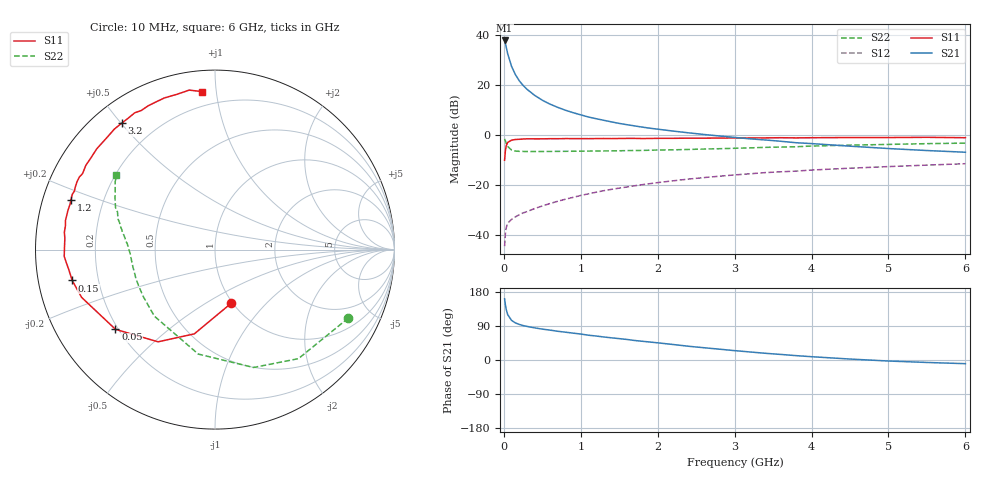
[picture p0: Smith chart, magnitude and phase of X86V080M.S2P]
! SIEMENS Small Signal Semiconductors
! BFP136W
! Si NPN RF Bipolar Junction Transistor in SOT343
! VCE = 6 V  IC = 80 mA
! Common Emitter S-Parameters:  September  1994
# GHz  S  MA  R  50
!  f  S11  S21  S12  S22
! GHz  MAG  ANG  MAG  ANG  MAG  ANG  MAG  ANG
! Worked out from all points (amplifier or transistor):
!   40 points, 10 MHz to 6 GHz, reference 50 ohm
!   highest |S21| = 37.9 dB at 10 MHz (marker M1)
!   |S21| within 3 dB of that: start of sweep to 33.25 MHz
!   unconditionally stable (mu >= 1): 655 MHz to 2.949 GHz
!   at 200 MHz: K = 0.63, MSG = 26.9 dB, |S12| = -32.0 dB
!   at 1.5 GHz: K = 1.10, MAG = 11.1 dB, |S12| = -21.3 dB
!   at 6 GHz: K = 0.96, MSG = 2.3 dB, |S12| = -11.5 dB
!   S11 on the Smith chart (normalised r, x): 10 MHz: 0.98, -0.65; 50 MHz: 0.19, -0.34; 150 MHz: 0.10, -0.11; 1.2 GHz: 0.08, +0.17; 3.2 GHz: 0.08, +0.50; 6 GHz: 0.11, +0.91
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0.01  0.3125 -73.3  78.95 161.4  0.0059 70.5  0.8351 -27.2
0.02  0.4834 -103.8  68.69 145.7  0.0105 59.0  0.7649 -52.6
0.03  0.6039 -121.7  58.87 134.2  0.0137 51.8  0.691 -71.9
0.05  0.7104 -141.3  42.74 119.8  0.017 40.3  0.5895 -99.1
0.1  0.7895 -160.3  23.93 104.6  0.0203 34.8  0.5017 -132.3
0.15  0.8138 -167.8  16.34 97.9  0.0228 37.2  0.4777 -146.8
0.2  0.8215 -171.9  12.3 93.9  0.0252 38.9  0.471 -154.7
0.25  0.8322 -175.2  9.936 90.9  0.0274 41.1  0.4693 -159.8
0.3  0.8409 -177.4  8.307 88.7  0.0291 42.6  0.467 -163.2
0.4  0.8385 178.8  6.261 84.8  0.0335 46.3  0.4673 -167.8
0.5  0.839 175.6  4.994 81.5  0.0378 49.5  0.468 -170.9
0.6  0.8448 173.5  4.169 78.9  0.0423 51.2  0.4691 -172.9
0.7  0.8437 170.8  3.594 75.8  0.0469 53.7  0.4704 -174.4
0.9  0.8477 167.1  2.811 70.9  0.0562 55.7  0.473 -177.1
1.1  0.8462 162.6  2.3 65.4  0.0662 57.0  0.4765 -178.8
1.2  0.849 161.1  2.125 63.3  0.0713 57.4  0.4791 -179.6
1.7  0.8572 151.9  1.525 51.5  0.096 56.4  0.4893 176.4
2.2  0.8597 143.5  1.201 40.9  0.1207 53.5  0.505 172.8
3.2  0.8755 126.5  0.839 21.2  0.167 45.1  0.5523 164.3
4.5  0.8908 108.6  0.598 2.5  0.2162 33.8  0.6269 152.7
5.5  0.9002 99.2  0.489 -6.5  0.2494 25.8  0.6719 145.9
6  0.8835 94.8  0.452 -9.7  0.2661 21.6  0.6884 142.9
